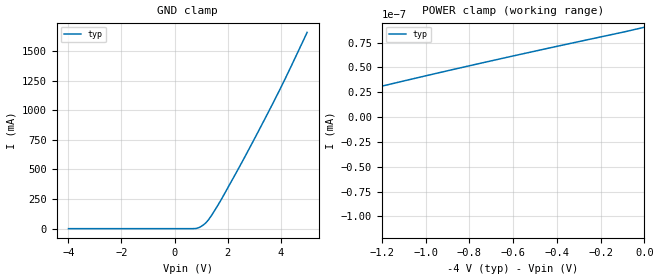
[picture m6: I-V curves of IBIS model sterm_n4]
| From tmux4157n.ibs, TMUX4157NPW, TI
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| sterm_n4
[Model]   sterm_n4
Model_type   Terminator
|   typ   min   max
C_comp   6.976543e-12   NA   NA
[Voltage Range]   -4   NA   NA
[Temperature Range]   27   NA   NA
[Power Clamp Reference]   -4   NA   NA
[GND Clamp Reference]   0   NA   NA
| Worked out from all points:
|   POWER clamp passes 1 mA (typ) near -4.76 V on its own axis
[GND Clamp]
|   Voltage   I(typ)   I(min)   I(max)
-4V       -150.7pA   NA         NA
727.3mV   478.2uA    NA         NA
909.1mV   7.91mA     NA         NA
1.091V    31.9mA     NA         NA
1.273V    72.66mA    NA         NA
1.545V    164.6mA    NA         NA
1.818V    268mA      NA         NA
2.636V    599.7mA    NA         NA
3.909V    1.146A     NA         NA
5V        1.656A     NA         NA
[POWER Clamp]
|   Voltage   I(typ)   I(min)   I(max)
-9V       -1.814A    NA         NA
-3.636V   -122pA     NA         NA
-3.545V   -115.2pA   NA         NA
-3.182V   -88.96pA   NA         NA
-2.727V   -58.24pA   NA         NA
-2.273V   -29.57pA   NA         NA
-1.818V   -2.744pA   NA         NA
-1V       41.51pA    NA         NA
0V        90.47pA    NA         NA
